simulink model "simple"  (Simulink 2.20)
settings: Solver=ode45  StartTime=0.0  StopTime=10.0  RelTol=1e-3  AbsTol=1e-6
libraries: simulink x1

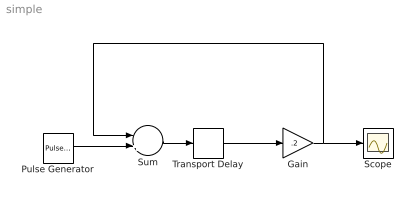
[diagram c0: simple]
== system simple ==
  Gain : Gain  Gain=.2
  Pulse Generator : simulink/Sources/Pulse Generator  period=1000  duty=50  amplitude=20  start=2
  Scope : Scope
  Sum : Sum  Inputs=-+
  Transport Delay : TransportDelay  DelayTime=.07  InitialInput=0  BufferSize=1024
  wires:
  Pulse Generator/1 -> Sum/2
  Sum/1 -> Transport Delay/1
  Transport Delay/1 -> Gain/1
  Gain/1 -> Scope/1, Sum/1
